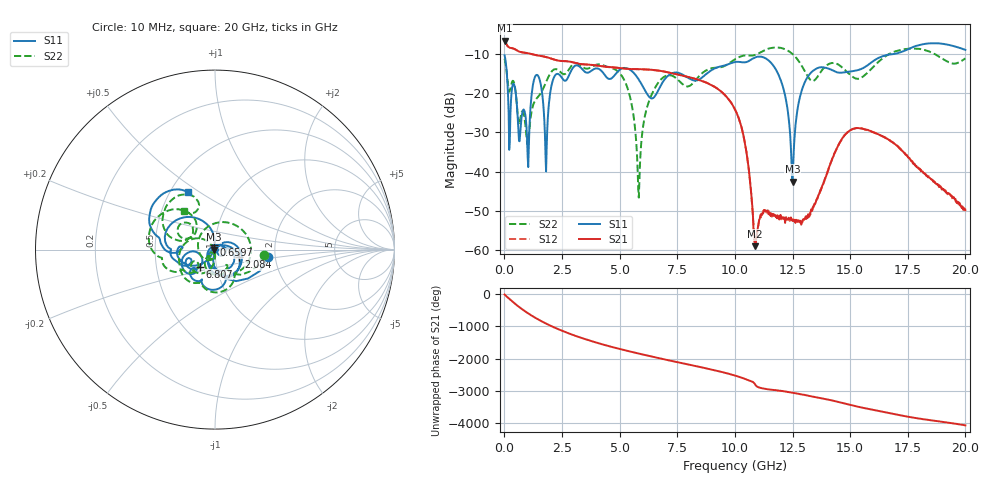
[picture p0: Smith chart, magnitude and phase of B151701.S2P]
!  2-Port S-parameters saved by WinCal
! VAR MeasName=S-Parameters (CALIBRATED_DATA) read from VNA (N5244A)
! VAR MeasDate=2015-12-24 19:07:55
! VAR NAME=B151701
! VAR FILENAME=B151701.S2P
! VAR DATE=2015-12-24 19:07:55
! VAR PHYS_PORTS=1,3
# Hz S DB R 50
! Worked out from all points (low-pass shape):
!   801 points, 10 MHz to 20 GHz, reference 50 ohm
!   highest |S21| = -6.66 dB at 10 MHz (marker M1); lowest = -59.0 dB at 10.88 GHz (marker M2)
!   |S21| within 3 dB of the highest: start of sweep to 756.3 MHz
!   lowest |S11| = -42.5 dB at 12.5 GHz (marker M3), VSWR 1.02, Z = 49.3 - j0.0538 ohm
!   |S11| at or under -10 dB: start of sweep to 16.97 GHz
!   |S22| runs from -46.6 to -8.4 dB; largest |S21 - S12| = 0.00096
!   S11 on the Smith chart (normalised r, x): 10 MHz: 1.84, -0.17; 659.7 MHz: 0.99, +0.05; 2.084 GHz: 1.30, -0.11; 6.807 GHz: 0.83, -0.16; 20 GHz: 0.61, +0.45
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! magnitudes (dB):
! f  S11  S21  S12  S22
! 10 MHz  -10.4  -6.7  -6.6  -11.3
! 209.9 MHz  -34.5  -8.4  -8.4  -19.7
! 409.8 MHz  -17.7  -8.7  -8.7  -17.2
! 659.7 MHz  -32.3  -9.5  -9.5  -27.6
! 1.034 GHz  -38.9  -9.9  -9.9  -32.3
! 1.409 GHz  -15.4  -10.4  -10.4  -21.3
! 1.809 GHz  -40.0  -10.9  -10.9  -17.2
! 2.084 GHz  -17.1  -11.4  -11.4  -14.3
! 3.358 GHz  -13.8  -12.7  -12.7  -13.2
! 5.157 GHz  -13.7  -13.8  -13.8  -16.3
! 5.832 GHz  -16.6  -14.0  -14.0  -46.6
! 6.682 GHz  -19.3  -14.3  -14.3  -17.3
! 6.807 GHz  -17.9  -14.4  -14.4  -16.5
! 10.01 GHz  -12.1  -24.2  -24.2  -11.4
! 10.48 GHz  -12.2  -34.2  -34.2  -10.4
! 10.88 GHz  -11.0  -59.0  -58.1  -10.3
! 11.95 GHz  -16.2  -51.7  -51.2  -8.5
! 12.5 GHz  -42.5  -52.5  -53.0  -10.1
! 13.35 GHz  -14.5  -50.0  -49.7  -17.0
! 14.85 GHz  -14.7  -30.2  -30.2  -14.6
! 16.68 GHz  -10.2  -31.9  -31.9  -10.1
! 20 GHz  -9.0  -49.8  -49.2  -11.2
